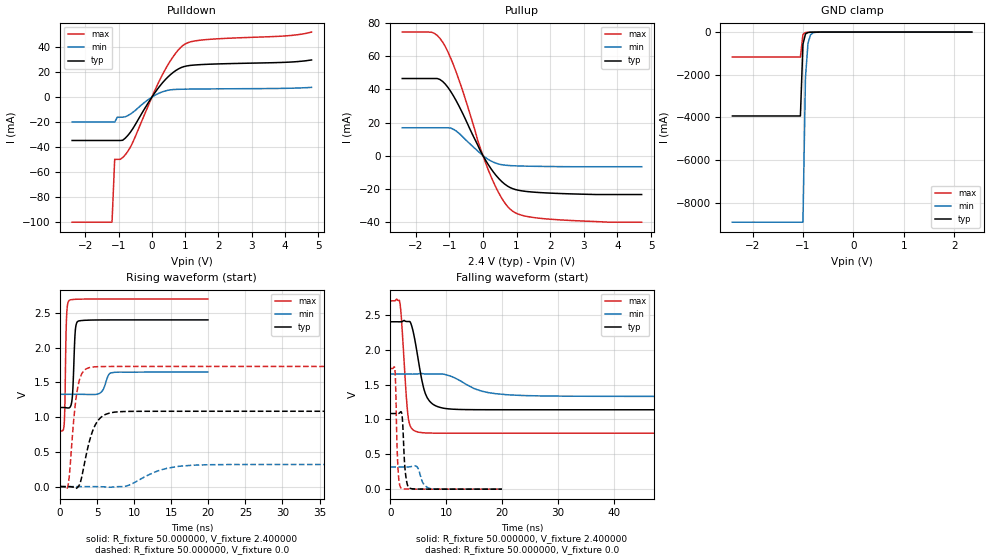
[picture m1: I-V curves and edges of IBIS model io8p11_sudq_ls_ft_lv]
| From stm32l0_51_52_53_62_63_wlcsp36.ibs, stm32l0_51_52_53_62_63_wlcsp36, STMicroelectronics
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|   Model io8p11_sudq_ls_ft_lv
[Model]  io8p11_sudq_ls_ft_lv
Model_type I/O
Polarity   Non-Inverting
Enable   Active-Low
Vinl =   0.720000V
Vinh =   1.680000V
Vmeas =  1.200000V
Cref =   50.000000pF
Rref =   100.000000M
Vref =   0.0V
C_comp   2.317700pF   2.286600pF   2.350000pF
[Temperature Range]   25.000000   0.125000k   -40.000000
[Pullup Reference]   2.400000V   1.650000V   2.700000V
[Pulldown Reference]   0.0V   0.0V   0.0V
[POWER Clamp Reference]   2.400000V   1.650000V   2.700000V
[GND Clamp Reference]   0.0V   0.0V   0.0V
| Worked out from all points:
|   slope of the pulldown table from 0 to 0.36 V, typ, clamps not added: 28.4 ohm
|   slope of the pullup table from 0 to 0.36 V, typ, clamps not added: 32.2 ohm
|   GND clamp passes 1 mA (typ) near -0.65 V on its own axis
|   rising waveform, R_fixture 50.000000, V_fixture 2.400000: 20-80 % time 278ps typ, 654ps min, 187ps max; typ from 1.14 V to 2.4 V
|   rising waveform, R_fixture 50.000000, V_fixture 0.0: 20-80 % time 1.58ns typ, 4ns min, 920ps max; typ from 0 V to 1.08 V
|   falling waveform, R_fixture 50.000000, V_fixture 2.400000: 20-80 % time 1.81ns typ, 5.27ns min, 912ps max; typ from 2.4 V to 1.14 V
|   falling waveform, R_fixture 50.000000, V_fixture 0.0: 20-80 % time 461ps typ, 889ps min, 359ps max; typ from 1.08 V to 0 V
[Pulldown]
|Voltage   I(typ)   I(min)   I(max)
-2.4V     -34.7mA    -20mA      -100mA
-1.2V     -34.7mA    -20mA      -100mA
-1.12V    -34.7mA    -20mA      -49.77mA
-1.04V    -34.7mA    -16.07mA   -49.77mA
-880mV    -34.55mA   -16.07mA   -48.41mA
-720mV    -30.52mA   -14.75mA   -43.24mA
-80mV     -3.3mA     -1.425mA   -4.982mA
320mV     11.47mA    4.218mA    18.08mA
640mV     19.72mA    5.982mA    32.34mA
960mV     24.32mA    6.291mA    41.77mA
1.52V     26.01mA    6.471mA    45.64mA
4.8V      29.64mA    7.741mA    51.92mA
[Pullup]
|Voltage   I(typ)   I(min)   I(max)
-2.4V     46.57mA    16.84mA    74.62mA
-1.52V    46.57mA    16.84mA    74.5mA
-1.2V     44.83mA    16.84mA    68.61mA
-800mV    33.29mA    14.93mA    50.64mA
-480mV    20.19mA    8.905mA    31.39mA
-160mV    6.586mA    2.887mA    9.467mA
240mV     -7.917mA   -3.247mA   -12.65mA
560mV     -15.67mA   -5.487mA   -25.76mA
880mV     -19.92mA   -6.092mA   -33.51mA
1.28V     -21.61mA   -6.351mA   -36.61mA
1.92V     -22.56mA   -6.557mA   -38.27mA
4.72V     -23.5mA    -6.7mA     -40.2mA
[GND_clamp]
|Voltage   I(typ)   I(min)   I(max)
-2.4V     -3.929A    -8.905A    -1.166A
-1.05V    -3.929A    -8.905A    -1.166A
-1V       -574.5mA   -8.905A    -109.1mA
-950mV    -90.02mA   -2.146A    -18.55mA
-900mV    -18.41mA   -523.6mA   -9.049mA
-850mV    -6.764mA   -130.9mA   -6.579mA
-800mV    -4.027mA   -34.58mA   -4.859mA
-600mV    -514.5uA   -843.4uA   -496.4uA
2.35V     0A         0A         0A
[POWER_clamp]
|Voltage   I(typ)   I(min)   I(max)
-2.4V     0A         0A         0A
0V        0A         0A         0A
[Ramp]
| variable   typ   min   max
dV/dt_r  0.65070/1.57846n   0.19118/3.99575n   1.03800/0.91475n
dV/dt_f  0.75696/1.80828n   0.18918/5.26371n   1.13786/0.91056n
R_load = 50.000000
[Rising Waveform]
R_fixture= 50.000000
V_fixture= 2.400000
V_fixture_min= 1.650000
V_fixture_max= 2.700000
|time   V(typ)   V(min)   V(max)
0s        1.139V     1.329V     802.5mV
560.6ps   1.138V     1.329V     920.4mV
840.8ps   1.135V     1.329V     2.378V
1.201ns   1.133V     1.329V     2.679V
1.642ns   1.29V      1.329V     2.693V
2.042ns   2.242V     1.329V     2.696V
2.402ns   2.38V      1.329V     2.698V
5.405ns   2.399V     1.348V     2.7V
7.087ns   2.4V       1.642V     2.7V
19.94ns   2.4V       1.65V      2.7V
[Rising Waveform]
R_fixture= 50.000000
V_fixture= 0.0
V_fixture_min= 0.0
V_fixture_max= 0.0
|time   V(typ)   V(min)   V(max)
0s        -3.073uV   4.597uV    228.3uV
1.001ns   110.4uV    1.131uV    -14.55mV
1.251ns   -727.1uV   -1.748uV   171.6mV
2.002ns   -17.33mV   -4.251uV   1.145V
2.377ns   -8.018mV   11.54uV    1.429V
4.004ns   674.6mV    87.44uV    1.714V
5.506ns   997mV      -1.925mV   1.728V
8.133ns   1.079V     -323.7uV   1.73V
17.89ns   1.085V     307.8mV    1.73V
62.31ns   1.085V     318.6mV    1.73V
[Falling Waveform]
R_fixture= 50.000000
V_fixture= 2.400000
V_fixture_min= 1.650000
V_fixture_max= 2.700000
|time   V(typ)   V(min)   V(max)
0s        2.4V       1.65V      2.7V
1.752ns   2.4V       1.65V      2.66V
3.128ns   2.404V     1.65V      1.08V
3.629ns   2.387V     1.65V      894.1mV
4.505ns   2.09V      1.65V      830.4mV
5.631ns   1.567V     1.658V     810.6mV
6.381ns   1.348V     1.652V     806.4mV
9.384ns   1.163V     1.65V      802.8mV
21.02ns   1.139V     1.353V     802.5mV
62.31ns   1.139V     1.329V     802.5mV
[Falling Waveform]
R_fixture= 50.000000
V_fixture= 0.0
V_fixture_min= 0.0
V_fixture_max= 0.0
|time   V(typ)   V(min)   V(max)
0s        1.085V     318.6mV    1.73V
840.8ps   1.085V     318.6mV    1.709V
1.361ns   1.084V     318.6mV    324.8mV
1.922ns   1.111V     318.6mV    14.52mV
2.202ns   961.9mV    318.6mV    3.937mV
2.683ns   249.1mV    318.3mV    2.132mV
3.403ns   17.82mV    320mV      1.329mV
4.725ns   1.802mV    325.3mV    585.8uV
7.207ns   455.9uV    6.824mV    264.2uV
19.94ns   -3.073uV   4.597uV    228.3uV
